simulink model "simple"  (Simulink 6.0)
settings: Solver=ode45  StartTime=0.0  StopTime=10.0  RelTol=1e-3
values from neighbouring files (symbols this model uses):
  tmp2 = [isempty(r0r2clk) isempty(r1r3clk) isempty(la) isempty(ld)  	      isempty(ra0) isempty(ra1) isempty(ra2) isempty(ra3) isempty(rc0)  	      isempty(rc1) isempty(rc2) isempty(rc3) isempty(rd0) isempty(rd1)  	      isempty(rd2) isempty(rd3)]    [createucf_fromvhdl.m]
undefined symbols (not defined in the file or in its folder): Bit, g, Location, Lower, Width, XP, XRCIIPro
libraries: xbsIndex_r3 x21, ADlibrary x4

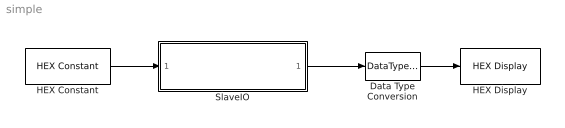
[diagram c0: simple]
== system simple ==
  Data Type Conversion : DataTypeConversion  OutDataTypeMode=double
  HEX Constant : ADlibrary/Miscellaneous/HEX Constant  value=1234ABCD
  HEX Display : ADlibrary/Miscellaneous/HEX Display
  SlaveIO : Subsystem
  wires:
  HEX Constant/1 -> SlaveIO/1(Vector Input)
  SlaveIO/1(Vector Output) -> Data Type Conversion/1
  Data Type Conversion/1 -> HEX Display/1

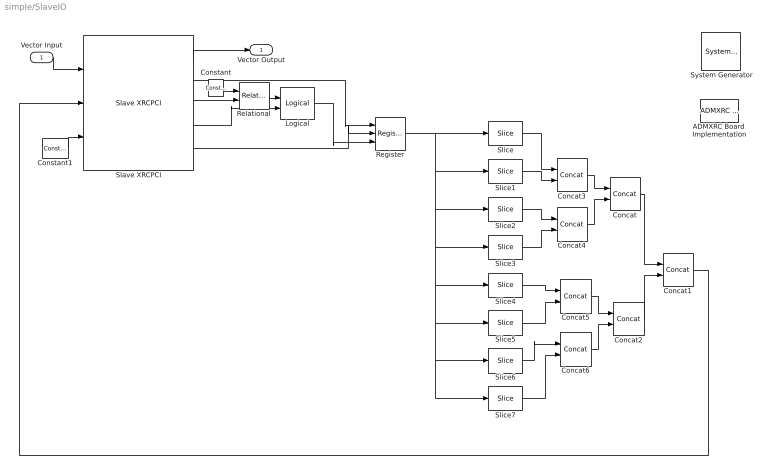
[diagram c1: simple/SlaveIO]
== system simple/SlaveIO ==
  Vector Input : Inport  Port=1  LatchInput=off
  " System Generator" : xbsIndex_r3/ System Generator  Tag=genX  xilinxfamily=Virtex2P  part=xc2vp70  speed=-6  package=ff1704  synthesis_tool=Synplify Pro  directory=g:/tmp2  testbench=off  simulink_period=1  sysclk_period=10  incr_netlist=off  trim_vbits=According to Block Masks  dbl_ovrd=According to Block Masks  core_generation=According to Block Masks  run_coregen=off  deprecated_control=off  eval_field=0
  ADMXRC Board  Implementation : ADlibrary/Miscellaneous/ADMXRC Board  Implementation  board=XRCIIPro(XP)  run_synth=on  make_clean=off  lvds_io_std=3.3v  clock_source=MCLK
  Concat{,1..6} (7 alike) : xbsIndex_r3/Concat  num_inputs=2  explicit_period=off  period=1  dbl_ovrd=off
  Constant : xbsIndex_r3/Constant  const=0  arith_type=Unsigned  n_bits=22  bin_pt=0  explicit_period=off  period=1  dbl_ovrd=off
  Constant1 : xbsIndex_r3/Constant  const=1  arith_type=Unsigned  n_bits=1  bin_pt=0  explicit_period=on  period=1  dbl_ovrd=off
  Logical : xbsIndex_r3/Logical  logical_function=AND  inputs=2  precision=Full  arith_type=Unsigned  n_bits=8  bin_pt=2  align_bp=on  latency=0  explicit_period=off  period=1  en=off  dbl_ovrd=off  show_param=off
  Register : xbsIndex_r3/Register  init=0  reg_only_valid=off  explicit_period=off  period=1  rst=on  en=on  out_en=off  dbl_ovrd=off  show_param=off
  Relational : xbsIndex_r3/Relational  mode=a=b  latency=0  explicit_period=off  period=1  en=off  dbl_ovrd=off  show_param=off
  Slave XRCPCI : ADlibrary/PCI/Slave XRCPCI  no_inputs=1  no_outputs=1  circuit_lag=1  decode_delay=0
  Slice : xbsIndex_r3/Slice  mode=Lower Bit Location + Width  nbits=4  bit1=0  base1=MSB of Input  bit0=0  base0=LSB of Input  boolean_output=off  explicit_period=off  period=1  dbl_ovrd=off
  Slice1 : xbsIndex_r3/Slice  mode=Lower Bit Location + Width  nbits=4  bit1=0  base1=MSB of Input  bit0=4  base0=LSB of Input  boolean_output=off  explicit_period=off  period=1  dbl_ovrd=off
  Slice2 : xbsIndex_r3/Slice  mode=Lower Bit Location + Width  nbits=4  bit1=0  base1=MSB of Input  bit0=8  base0=LSB of Input  boolean_output=off  explicit_period=off  period=1  dbl_ovrd=off
  Slice3 : xbsIndex_r3/Slice  mode=Lower Bit Location + Width  nbits=4  bit1=0  base1=MSB of Input  bit0=12  base0=LSB of Input  boolean_output=off  explicit_period=off  period=1  dbl_ovrd=off
  Slice4 : xbsIndex_r3/Slice  mode=Lower Bit Location + Width  nbits=4  bit1=0  base1=MSB of Input  bit0=16  base0=LSB of Input  boolean_output=off  explicit_period=off  period=1  dbl_ovrd=off
  Slice5 : xbsIndex_r3/Slice  mode=Lower Bit Location + Width  nbits=4  bit1=0  base1=MSB of Input  bit0=20  base0=LSB of Input  boolean_output=off  explicit_period=off  period=1  dbl_ovrd=off
  Slice6 : xbsIndex_r3/Slice  mode=Lower Bit Location + Width  nbits=4  bit1=0  base1=MSB of Input  bit0=24  base0=LSB of Input  boolean_output=off  explicit_period=off  period=1  dbl_ovrd=off
  Slice7 : xbsIndex_r3/Slice  mode=Lower Bit Location + Width  nbits=4  bit1=0  base1=MSB of Input  bit0=28  base0=LSB of Input  boolean_output=off  explicit_period=off  period=1  dbl_ovrd=off
  Vector Output : Outport
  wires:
  Slave XRCPCI/1 -> Vector Output/1
  Vector Input/1 -> Slave XRCPCI/1
  Concat3/1 -> Concat/1
  Concat4/1 -> Concat/2
  Concat5/1 -> Concat2/1
  Concat6/1 -> Concat2/2
  Slice/1 -> Concat3/1
  Slice1/1 -> Concat3/2
  Slice2/1 -> Concat4/1
  Slice3/1 -> Concat4/2
  Slice4/1 -> Concat5/1
  Slice5/1 -> Concat5/2
  Slice6/1 -> Concat6/1
  Slice7/1 -> Concat6/2
  Concat/1 -> Concat1/1
  Logical/1 -> Register/3
  Register/1 -> Slice/1, Slice7/1, Slice6/1, Slice5/1, Slice4/1, Slice3/1, Slice2/1, Slice1/1
  Concat2/1 -> Concat1/2
  Constant1/1 -> Slave XRCPCI/3
  Constant/1 -> Relational/1
  Slave XRCPCI/3 -> Relational/2
  Relational/1 -> Logical/1
  Slave XRCPCI/4 -> Logical/2
  Slave XRCPCI/5 -> Register/2
  Concat1/1 -> Slave XRCPCI/2
  Slave XRCPCI/2 -> Register/1
